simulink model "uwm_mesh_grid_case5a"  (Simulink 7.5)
settings: Solver=ode45  StartTime=0.0  StopTime=3.0  RelTol=1e-4
undefined symbols (not defined in the file or in its folder): D1, Delta, dfilt, DiscIntNeverNeededParam, Discrete, no, powergui, steady, ZData
libraries: powerlib x259, powerlib_extras x68, dsparch4 x11
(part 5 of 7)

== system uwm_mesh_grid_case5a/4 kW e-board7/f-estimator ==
  v : Inport
  Constant : Constant  Value=60  OutDataType=fixdt(1, 16)  OutScaling=2^0
  Fcn : Fcn  Expr=sin(2*pi*u[1])
  Filter1 : dsparch4/Biquad Filter  Tag=BlockMethodSubSystem  DialogController=dspdialog.BiquadFilter  DialogControllerArgs=DataTag8  IIRFiltStruct=Direct form II  CoeffSource=Specify via dialog  BiQuadCoeffs=[1 -1.36 1 1 -1.78 0.87;1 1 0 1 -0.85 0]  a0Flag=Warning  IC=0  ICnum=0  ICden=0  denAccumFracLength=30  denProdOutputFracLength=30  secondMemoryFracLength=15  roundingMode=Floor  overflowMode=off  ScaleValues=[0.05;0.23;1]  optimizeScaleValues=on  ScaleValueMode=Specify via input port (g)  scaleValueFracLength=14  FilterSource=Specify via dialog  dfiltObjectName=dfilt.df2tsos([1 0.3 0.4],[1 0.1 0.2])
  Gain : Gain  Gain=1/150  ParameterDataType=fixdt(1, 16)  ParameterScaling=2^0  OutDataType=fixdt(1, 16)  OutScaling=2^0  SampleTime=dt
  Product : Product  OutDataType=fixdt(1, 16)  OutScaling=2^0
  Scope : Scope
  Sum : Sum  Inputs=|++  OutDataType=fixdt(1, 16)  OutScaling=2^0
  modulo discrete integrator : Subsystem  mask{dt=dt}
      mask prompts: dt "sample time"
  w : Outport  OutDataType=fixdt(1, 16)  OutScaling=2^0
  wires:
  Gain/1 -> Product/1
  v/1 -> Gain/1
  Filter1/1 -> Sum/1, Scope/1
  Product/1 -> Filter1/1
  Sum/1 -> w/1, modulo discrete integrator/1(In1)
  modulo discrete integrator/1(Out1) -> Fcn/1
  Constant/1 -> Sum/2
  Fcn/1 -> Product/2

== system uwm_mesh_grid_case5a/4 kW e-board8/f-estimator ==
  v : Inport
  Constant : Constant  Value=60  OutDataType=fixdt(1, 16)  OutScaling=2^0
  Fcn : Fcn  Expr=sin(2*pi*u[1])
  Filter1 : dsparch4/Biquad Filter  Tag=BlockMethodSubSystem  DialogController=dspdialog.BiquadFilter  DialogControllerArgs=DataTag9  IIRFiltStruct=Direct form II  CoeffSource=Specify via dialog  BiQuadCoeffs=[1 -1.36 1 1 -1.78 0.87;1 1 0 1 -0.85 0]  a0Flag=Warning  IC=0  ICnum=0  ICden=0  denAccumFracLength=30  denProdOutputFracLength=30  secondMemoryFracLength=15  roundingMode=Floor  overflowMode=off  ScaleValues=[0.05;0.23;1]  optimizeScaleValues=on  ScaleValueMode=Specify via input port (g)  scaleValueFracLength=14  FilterSource=Specify via dialog  dfiltObjectName=dfilt.df2tsos([1 0.3 0.4],[1 0.1 0.2])
  Gain : Gain  Gain=1/150  ParameterDataType=fixdt(1, 16)  ParameterScaling=2^0  OutDataType=fixdt(1, 16)  OutScaling=2^0  SampleTime=dt
  Product : Product  OutDataType=fixdt(1, 16)  OutScaling=2^0
  Scope : Scope
  Sum : Sum  Inputs=|++  OutDataType=fixdt(1, 16)  OutScaling=2^0
  modulo discrete integrator : Subsystem  mask{dt=dt}
      mask prompts: dt "sample time"
  w : Outport  OutDataType=fixdt(1, 16)  OutScaling=2^0
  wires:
  Gain/1 -> Product/1
  v/1 -> Gain/1
  Filter1/1 -> Sum/1, Scope/1
  Product/1 -> Filter1/1
  Sum/1 -> w/1, modulo discrete integrator/1(In1)
  modulo discrete integrator/1(Out1) -> Fcn/1
  Constant/1 -> Sum/2
  Fcn/1 -> Product/2

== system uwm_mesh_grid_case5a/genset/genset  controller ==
  wr : Inport
  Vabc : Inport  Port=2
  Iabc : Inport  Port=3
  Preq : Inport  Port=4
  Ereq1 : Inport  Port=5
  Gain : Gain  ParameterDataType=fixdt(1, 16)  ParameterScaling=2^0  OutDataType=fixdt(1, 16)  OutScaling=2^0
  P-w droop : Subsystem
  PVQ computation : Subsystem
  Q-E droop : Subsystem
  exciter : Subsystem
  ic_engine gpvernor : Subsystem
  Pmech : Outport
  Vf : Outport  Port=2
  w : Outport  Port=3
  Pmm : Outport  Port=4
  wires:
  P-w droop/1(w) -> w/1, ic_engine gpvernor/3(w)
  PVQ computation/1(P_pu) -> P-w droop/2(P), ic_engine gpvernor/2(Pmeas)
  PVQ computation/3(Q_pu) -> Q-E droop/2(Q)
  Q-E droop/1(Vpk) -> exciter/2(Ef_mcd_wr)
  ic_engine gpvernor/1(Pmech) -> Pmech/1
  Vabc/1 -> PVQ computation/1(Vabc)
  Iabc/1 -> PVQ computation/2(Iabc)
  exciter/1(Ef) -> Vf/1
  Preq/1 -> P-w droop/1(P_req)
  Ereq1/1 -> Q-E droop/3(E_req)
  PVQ computation/2(Vt) -> Q-E droop/1(v_meas)
  Gain/1 -> ic_engine gpvernor/1(wr), exciter/1(wr)
  wr/1 -> Gain/1
  P-w droop/2(Pmm) -> Pmm/1

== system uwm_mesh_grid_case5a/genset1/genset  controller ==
  wr : Inport
  Vabc : Inport  Port=2
  Iabc : Inport  Port=3
  Preq : Inport  Port=4
  Ereq1 : Inport  Port=5
  Gain : Gain  ParameterDataType=fixdt(1, 16)  ParameterScaling=2^0  OutDataType=fixdt(1, 16)  OutScaling=2^0
  P-w droop : Subsystem
  PVQ computation : Subsystem
  Q-E droop : Subsystem
  exciter : Subsystem
  ic_engine gpvernor : Subsystem
  Pmech : Outport
  Vf : Outport  Port=2
  w : Outport  Port=3
  Pmm : Outport  Port=4
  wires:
  P-w droop/1(w) -> w/1, ic_engine gpvernor/3(w)
  PVQ computation/1(P_pu) -> P-w droop/2(P), ic_engine gpvernor/2(Pmeas)
  PVQ computation/3(Q_pu) -> Q-E droop/2(Q)
  Q-E droop/1(Vpk) -> exciter/2(Ef_mcd_wr)
  ic_engine gpvernor/1(Pmech) -> Pmech/1
  Vabc/1 -> PVQ computation/1(Vabc)
  Iabc/1 -> PVQ computation/2(Iabc)
  exciter/1(Ef) -> Vf/1
  Preq/1 -> P-w droop/1(P_req)
  Ereq1/1 -> Q-E droop/3(E_req)
  PVQ computation/2(Vt) -> Q-E droop/1(v_meas)
  Gain/1 -> ic_engine gpvernor/1(wr), exciter/1(wr)
  wr/1 -> Gain/1
  P-w droop/2(Pmm) -> Pmm/1

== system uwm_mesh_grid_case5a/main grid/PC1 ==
  Three-Phase Series RLC Branch3 : powerlib/Elements/Three-Phase Series RLC Branch  DialogController=POWERSYS.PowerSysDialog  PhysicalDomain=powersysdomain  SubClassName=unknown  LeftPortType=p1  RightPortType=p1  LConnTagsString=A|B|C  RConnTagsString=A|B|C  BranchType=RL  Resistance=R  Inductance=L  Capacitance=1/(336*2*pi*60)  Measurements=None
  A* : PMIOPort  Tag=PMCPort  Port=1  Side=Right
  B* : PMIOPort  Tag=PMCPort  Port=2  Side=Right
  C* : PMIOPort  Tag=PMCPort  Port=3  Side=Right
  A : PMIOPort  Tag=PMCPort  Port=4  Side=Left
  B : PMIOPort  Tag=PMCPort  Port=5  Side=Left
  C : PMIOPort  Tag=PMCPort  Port=6  Side=Left
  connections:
  A*/RConn1 -- Three-Phase Series RLC Branch3/LConn1
  B*/RConn1 -- Three-Phase Series RLC Branch3/LConn2
  C*/RConn1 -- Three-Phase Series RLC Branch3/LConn3
  Three-Phase Series RLC Branch3/RConn1 -- A/RConn1
  Three-Phase Series RLC Branch3/RConn2 -- B/RConn1
  Three-Phase Series RLC Branch3/RConn3 -- C/RConn1

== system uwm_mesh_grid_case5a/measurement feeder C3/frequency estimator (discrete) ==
  v : Inport
  Constant : Constant  Value=60  OutDataType=fixdt(1, 16)  OutScaling=2^0
  Fcn : Fcn  Expr=sin(2*pi*u[1])
  Filter1 : dsparch4/Biquad Filter  Tag=BlockMethodSubSystem  DialogController=dspdialog.BiquadFilter  DialogControllerArgs=DataTag10  IIRFiltStruct=Direct form II  CoeffSource=Specify via dialog  BiQuadCoeffs=[1 -1.36 1 1 -1.78 0.87;1 1 0 1 -0.85 0]  a0Flag=Warning  IC=0  ICnum=0  ICden=0  denAccumFracLength=30  denProdOutputFracLength=30  secondMemoryFracLength=15  roundingMode=Floor  overflowMode=off  ScaleValues=[0.05;0.23;1]  optimizeScaleValues=on  ScaleValueMode=Specify via input port (g)  scaleValueFracLength=14  FilterSource=Specify via dialog  dfiltObjectName=dfilt.df2tsos([1 0.3 0.4],[1 0.1 0.2])
  Gain : Gain  Gain=1/150  ParameterDataType=fixdt(1, 16)  ParameterScaling=2^0  OutDataType=fixdt(1, 16)  OutScaling=2^0  SampleTime=dt
  Product : Product  OutDataType=fixdt(1, 16)  OutScaling=2^0
  Scope : Scope
  Sum : Sum  Inputs=|++  OutDataType=fixdt(1, 16)  OutScaling=2^0
  modulo discrete integrator : Subsystem  mask{dt=dt}
      mask prompts: dt "sample time"
  w : Outport  OutDataType=fixdt(1, 16)  OutScaling=2^0
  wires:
  Fcn/1 -> Product/2
  Constant/1 -> Sum/2
  modulo discrete integrator/1(Out1) -> Fcn/1
  Sum/1 -> modulo discrete integrator/1(In1), w/1
  Product/1 -> Filter1/1
  Filter1/1 -> Scope/1, Sum/1
  v/1 -> Gain/1
  Gain/1 -> Product/1

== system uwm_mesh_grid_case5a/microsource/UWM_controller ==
  note: P
  note: Q
  v_meas : Inport
  i_meas : Inport  Port=2
  E_req : Inport  Port=3
  P_req : Inport  Port=4
  " pu convert P" : Gain  Gain=1/Sbase  ParameterDataType=sfix(16)  ParameterScaling=2^0  OutDataType=sfix(16)  OutScaling=2^0
  " pu convert S" : Gain  Gain=1/Sbase  ParameterDataType=sfix(16)  ParameterScaling=2^0  OutDataType=sfix(16)  OutScaling=2^0
  " pu convert V" : Gain  Gain=1/(Vbase/sqrt(3))  ParameterDataType=sfix(16)  ParameterScaling=2^0  OutDataType=sfix(16)  OutScaling=2^0
  3-phase  Instantaneous  Active & Reactive Power : powerlib_extras/Measurements/3-phase  Instantaneous  Active & Reactive Power  DialogController=POWERSYS.PowerSysDialog  SystemSampleTime=-1
  Demux : Demux  Outputs=2
  PI-Control : Subsystem
  RMS : Fcn  Expr=sqrt(u(1)*u(1)+u(2)*u(2)+u(3)*u(3))/sqrt(3)
  Sum : Sum  Inputs=|-+  OutDataType=sfix(16)  OutScaling=2^0
  Sum1 : Sum  Inputs=|+-  OutDataType=sfix(16)  OutScaling=2^0
  Sum2 : Sum  Inputs=+-|  OutDataType=sfix(16)  OutScaling=2^0
  Sum3 : Sum  Inputs=+++  OutDataType=sfix(16)  OutScaling=2^0
  Transfer Fcn : TransferFcn  Denominator=[.01 1]
  Transfer Fcn1 : TransferFcn  Denominator=[.01 1]
  Transfer Fcn2 : TransferFcn  Denominator=[.01 1]
  k : Gain  Gain=1/pi  ParameterDataType=sfix(16)  ParameterScaling=2^0  OutDataType=sfix(16)  OutScaling=2^0
  limiter : Subsystem
  mP droop : Gain  Gain=pi  ParameterDataType=sfix(16)  ParameterScaling=2^0  OutDataType=sfix(16)  OutScaling=2^0
  "mQ droop " : Gain  Gain=0.05  ParameterDataType=sfix(16)  ParameterScaling=2^0  OutDataType=sfix(16)  OutScaling=2^0
  w0 : Constant  Value=60*2*pi  OutDataType=fixdt(1, 16)  OutScaling=2^0
  Vpk : Outport
  w : Outport  Port=2
  Pmm : Outport  Port=3
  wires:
  Transfer Fcn2/1 -> " pu convert V"/1
  Transfer Fcn/1 -> " pu convert P"/1
  " pu convert P"/1 -> "mQ droop "/1
  Transfer Fcn1/1 -> " pu convert S"/1
  " pu convert S"/1 -> limiter/1(In1), Sum2/2
  i_meas/1 -> 3-phase  Instantaneous  Active & Reactive Power/2
  P_req/1 -> Sum2/1
  mP droop/1 -> Sum3/2
  limiter/1(Out1) -> Sum3/1, k/1
  w0/1 -> Sum3/3
  Sum2/1 -> mP droop/1
  Sum1/1 -> PI-Control/1(In1)
  Sum/1 -> Sum1/1
  "mQ droop "/1 -> Sum/1
  RMS/1 -> Transfer Fcn2/1
  Demux/2 -> Transfer Fcn/1
  Demux/1 -> Transfer Fcn1/1
  3-phase  Instantaneous  Active & Reactive Power/1 -> Demux/1
  v_meas/1 -> RMS/1, 3-phase  Instantaneous  Active & Reactive Power/1
  PI-Control/1(Out1) -> Vpk/1
  Sum3/1 -> w/1
  E_req/1 -> Sum/2
  " pu convert V"/1 -> Sum1/2
  k/1 -> Pmm/1

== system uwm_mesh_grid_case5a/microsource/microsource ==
  Vpk : Inport  OutDataType=fixdt(1, 16)  OutScaling=2^0
  w : Inport  Port=2  OutDataType=fixdt(1, 16)  OutScaling=2^0
  Demux : Demux  Outputs=3
  Ground2 : powerlib/Elements/Ground  DialogController=POWERSYS.PowerSysDialog  PhysicalDomain=powersysdomain  SubClassName=unknown  LeftPortType=p1  RightPortType=p1  LConnTagsString=a
  Integrator : Integrator
  Mux : Mux  Inputs=3
  Product : Product  OutDataType=sfix(16)  OutScaling=2^0
  Series RLC Branch : powerlib/Elements/Series RLC Branch  DialogController=POWERSYS.PowerSysDialog  PhysicalDomain=powersysdomain  SubClassName=unknown  LeftPortType=p1  RightPortType=p1  LConnTagsString=__new0  RConnTagsString=__new0  BranchType=C  Resistance=1  Inductance=1e-3  SetiL0=off  InitialCurrent=0  Capacitance=1e-8  Setx0=off  InitialVoltage=0  Measurements=None
  phaseA : powerlib/Electrical Sources/Controlled Voltage Source  DialogController=POWERSYS.PowerSysDialog  SystemSampleTime=-1  Initialize=on  Source_Type=AC  Amplitude=0  Phase=0  Frequency=0  Measurements=None
  phaseB : powerlib/Electrical Sources/Controlled Voltage Source  DialogController=POWERSYS.PowerSysDialog  SystemSampleTime=-1  Initialize=on  Source_Type=AC  Amplitude=0  Phase=0  Frequency=0  Measurements=None
  phaseC : powerlib/Electrical Sources/Controlled Voltage Source  DialogController=POWERSYS.PowerSysDialog  SystemSampleTime=-1  Initialize=on  Source_Type=AC  Amplitude=0  Phase=0  Frequency=0  Measurements=None
  v_A : Fcn  Expr=cos(u)
  v_B : Fcn  Expr=cos(u-2*pi/3)
  v_C : Fcn  Expr=cos(u+2*pi/3)
  Va : PMIOPort  Tag=PMCPort  Port=1  Side=Right
  Vb : PMIOPort  Tag=PMCPort  Port=2  Side=Right
  Vc : PMIOPort  Tag=PMCPort  Port=3  Side=Right
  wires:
  Product/1 -> Demux/1
  Vpk/1 -> Product/1
  Mux/1 -> Product/2
  w/1 -> Integrator/1
  Integrator/1 -> v_A/1, v_B/1, v_C/1
  v_A/1 -> Mux/1
  v_B/1 -> Mux/2
  v_C/1 -> Mux/3
  Demux/1 -> phaseA/1
  Demux/2 -> phaseB/1
  Demux/3 -> phaseC/1
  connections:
  Vb/RConn1 -- phaseB/RConn1 -- phaseA/LConn1
  Va/RConn1 -- phaseC/LConn1 -- phaseA/RConn1
  Vc/RConn1 -- phaseC/RConn1
  Series RLC Branch/RConn1 -- Ground2/LConn1
  Series RLC Branch/LConn1 -- phaseB/LConn1

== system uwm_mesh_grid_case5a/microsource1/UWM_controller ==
  note: P
  note: Q
  v_meas : Inport
  i_meas : Inport  Port=2
  E_req : Inport  Port=3
  P_req : Inport  Port=4
  " pu convert P" : Gain  Gain=1/Sbase  ParameterDataType=sfix(16)  ParameterScaling=2^0  OutDataType=sfix(16)  OutScaling=2^0
  " pu convert S" : Gain  Gain=1/Sbase  ParameterDataType=sfix(16)  ParameterScaling=2^0  OutDataType=sfix(16)  OutScaling=2^0
  " pu convert V" : Gain  Gain=1/(Vbase/sqrt(3))  ParameterDataType=sfix(16)  ParameterScaling=2^0  OutDataType=sfix(16)  OutScaling=2^0
  3-phase  Instantaneous  Active & Reactive Power : powerlib_extras/Measurements/3-phase  Instantaneous  Active & Reactive Power  DialogController=POWERSYS.PowerSysDialog  SystemSampleTime=-1
  Demux : Demux  Outputs=2
  PI-Control : Subsystem
  RMS : Fcn  Expr=sqrt(u(1)*u(1)+u(2)*u(2)+u(3)*u(3))/sqrt(3)
  Sum : Sum  Inputs=|-+  OutDataType=sfix(16)  OutScaling=2^0
  Sum1 : Sum  Inputs=|+-  OutDataType=sfix(16)  OutScaling=2^0
  Sum2 : Sum  Inputs=+-|  OutDataType=sfix(16)  OutScaling=2^0
  Sum3 : Sum  Inputs=+++  OutDataType=sfix(16)  OutScaling=2^0
  Transfer Fcn : TransferFcn  Denominator=[.01 1]
  Transfer Fcn1 : TransferFcn  Denominator=[.01 1]
  Transfer Fcn2 : TransferFcn  Denominator=[.01 1]
  k : Gain  Gain=1/pi  ParameterDataType=sfix(16)  ParameterScaling=2^0  OutDataType=sfix(16)  OutScaling=2^0
  limiter : Subsystem
  mP droop : Gain  Gain=pi  ParameterDataType=sfix(16)  ParameterScaling=2^0  OutDataType=sfix(16)  OutScaling=2^0
  "mQ droop " : Gain  Gain=0.05  ParameterDataType=sfix(16)  ParameterScaling=2^0  OutDataType=sfix(16)  OutScaling=2^0
  w0 : Constant  Value=60*2*pi  OutDataType=fixdt(1, 16)  OutScaling=2^0
  Vpk : Outport
  w : Outport  Port=2
  Pmm : Outport  Port=3
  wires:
  Transfer Fcn2/1 -> " pu convert V"/1
  Transfer Fcn/1 -> " pu convert P"/1
  " pu convert P"/1 -> "mQ droop "/1
  Transfer Fcn1/1 -> " pu convert S"/1
  " pu convert S"/1 -> limiter/1(In1), Sum2/2
  i_meas/1 -> 3-phase  Instantaneous  Active & Reactive Power/2
  P_req/1 -> Sum2/1
  mP droop/1 -> Sum3/2
  limiter/1(Out1) -> Sum3/1, k/1
  w0/1 -> Sum3/3
  Sum2/1 -> mP droop/1
  Sum1/1 -> PI-Control/1(In1)
  Sum/1 -> Sum1/1
  "mQ droop "/1 -> Sum/1
  RMS/1 -> Transfer Fcn2/1
  Demux/2 -> Transfer Fcn/1
  Demux/1 -> Transfer Fcn1/1
  3-phase  Instantaneous  Active & Reactive Power/1 -> Demux/1
  v_meas/1 -> RMS/1, 3-phase  Instantaneous  Active & Reactive Power/1
  PI-Control/1(Out1) -> Vpk/1
  Sum3/1 -> w/1
  E_req/1 -> Sum/2
  " pu convert V"/1 -> Sum1/2
  k/1 -> Pmm/1

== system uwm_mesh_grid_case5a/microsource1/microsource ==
  Vpk : Inport  OutDataType=fixdt(1, 16)  OutScaling=2^0
  w : Inport  Port=2  OutDataType=fixdt(1, 16)  OutScaling=2^0
  Demux : Demux  Outputs=3
  Ground2 : powerlib/Elements/Ground  DialogController=POWERSYS.PowerSysDialog  PhysicalDomain=powersysdomain  SubClassName=unknown  LeftPortType=p1  RightPortType=p1  LConnTagsString=a
  Integrator : Integrator
  Mux : Mux  Inputs=3
  Product : Product  OutDataType=sfix(16)  OutScaling=2^0
  Series RLC Branch : powerlib/Elements/Series RLC Branch  DialogController=POWERSYS.PowerSysDialog  PhysicalDomain=powersysdomain  SubClassName=unknown  LeftPortType=p1  RightPortType=p1  LConnTagsString=__new0  RConnTagsString=__new0  BranchType=C  Resistance=1  Inductance=1e-3  SetiL0=off  InitialCurrent=0  Capacitance=1e-8  Setx0=off  InitialVoltage=0  Measurements=None
  phaseA : powerlib/Electrical Sources/Controlled Voltage Source  DialogController=POWERSYS.PowerSysDialog  SystemSampleTime=-1  Initialize=on  Source_Type=AC  Amplitude=0  Phase=0  Frequency=0  Measurements=None
  phaseB : powerlib/Electrical Sources/Controlled Voltage Source  DialogController=POWERSYS.PowerSysDialog  SystemSampleTime=-1  Initialize=on  Source_Type=AC  Amplitude=0  Phase=0  Frequency=0  Measurements=None
  phaseC : powerlib/Electrical Sources/Controlled Voltage Source  DialogController=POWERSYS.PowerSysDialog  SystemSampleTime=-1  Initialize=on  Source_Type=AC  Amplitude=0  Phase=0  Frequency=0  Measurements=None
  v_A : Fcn  Expr=cos(u)
  v_B : Fcn  Expr=cos(u-2*pi/3)
  v_C : Fcn  Expr=cos(u+2*pi/3)
  Va : PMIOPort  Tag=PMCPort  Port=1  Side=Right
  Vb : PMIOPort  Tag=PMCPort  Port=2  Side=Right
  Vc : PMIOPort  Tag=PMCPort  Port=3  Side=Right
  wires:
  Product/1 -> Demux/1
  Vpk/1 -> Product/1
  Mux/1 -> Product/2
  w/1 -> Integrator/1
  Integrator/1 -> v_A/1, v_B/1, v_C/1
  v_A/1 -> Mux/1
  v_B/1 -> Mux/2
  v_C/1 -> Mux/3
  Demux/1 -> phaseA/1
  Demux/2 -> phaseB/1
  Demux/3 -> phaseC/1
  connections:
  Vb/RConn1 -- phaseB/RConn1 -- phaseA/LConn1
  Va/RConn1 -- phaseC/LConn1 -- phaseA/RConn1
  Vc/RConn1 -- phaseC/RConn1
  Series RLC Branch/RConn1 -- Ground2/LConn1
  Series RLC Branch/LConn1 -- phaseB/LConn1

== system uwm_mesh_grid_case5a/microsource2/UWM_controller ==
  note: P
  note: Q
  v_meas : Inport
  i_meas : Inport  Port=2
  E_req : Inport  Port=3
  P_req : Inport  Port=4
  " pu convert P" : Gain  Gain=1/Sbase  ParameterDataType=sfix(16)  ParameterScaling=2^0  OutDataType=sfix(16)  OutScaling=2^0
  " pu convert S" : Gain  Gain=1/Sbase  ParameterDataType=sfix(16)  ParameterScaling=2^0  OutDataType=sfix(16)  OutScaling=2^0
  " pu convert V" : Gain  Gain=1/(Vbase/sqrt(3))  ParameterDataType=sfix(16)  ParameterScaling=2^0  OutDataType=sfix(16)  OutScaling=2^0
  3-phase  Instantaneous  Active & Reactive Power : powerlib_extras/Measurements/3-phase  Instantaneous  Active & Reactive Power  DialogController=POWERSYS.PowerSysDialog  SystemSampleTime=-1
  Demux : Demux  Outputs=2
  PI-Control : Subsystem
  RMS : Fcn  Expr=sqrt(u(1)*u(1)+u(2)*u(2)+u(3)*u(3))/sqrt(3)
  Sum : Sum  Inputs=|-+  OutDataType=sfix(16)  OutScaling=2^0
  Sum1 : Sum  Inputs=|+-  OutDataType=sfix(16)  OutScaling=2^0
  Sum2 : Sum  Inputs=+-|  OutDataType=sfix(16)  OutScaling=2^0
  Sum3 : Sum  Inputs=+++  OutDataType=sfix(16)  OutScaling=2^0
  Transfer Fcn : TransferFcn  Denominator=[.01 1]
  Transfer Fcn1 : TransferFcn  Denominator=[.01 1]
  Transfer Fcn2 : TransferFcn  Denominator=[.01 1]
  k : Gain  Gain=1/pi  ParameterDataType=sfix(16)  ParameterScaling=2^0  OutDataType=sfix(16)  OutScaling=2^0
  limiter : Subsystem
  mP droop : Gain  Gain=pi  ParameterDataType=sfix(16)  ParameterScaling=2^0  OutDataType=sfix(16)  OutScaling=2^0
  "mQ droop " : Gain  Gain=0.05  ParameterDataType=sfix(16)  ParameterScaling=2^0  OutDataType=sfix(16)  OutScaling=2^0
  w0 : Constant  Value=60*2*pi  OutDataType=fixdt(1, 16)  OutScaling=2^0
  Vpk : Outport
  w : Outport  Port=2
  Pmm : Outport  Port=3
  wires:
  Transfer Fcn2/1 -> " pu convert V"/1
  Transfer Fcn/1 -> " pu convert P"/1
  " pu convert P"/1 -> "mQ droop "/1
  Transfer Fcn1/1 -> " pu convert S"/1
  " pu convert S"/1 -> limiter/1(In1), Sum2/2
  i_meas/1 -> 3-phase  Instantaneous  Active & Reactive Power/2
  P_req/1 -> Sum2/1
  mP droop/1 -> Sum3/2
  limiter/1(Out1) -> Sum3/1, k/1
  w0/1 -> Sum3/3
  Sum2/1 -> mP droop/1
  Sum1/1 -> PI-Control/1(In1)
  Sum/1 -> Sum1/1
  "mQ droop "/1 -> Sum/1
  RMS/1 -> Transfer Fcn2/1
  Demux/2 -> Transfer Fcn/1
  Demux/1 -> Transfer Fcn1/1
  3-phase  Instantaneous  Active & Reactive Power/1 -> Demux/1
  v_meas/1 -> RMS/1, 3-phase  Instantaneous  Active & Reactive Power/1
  PI-Control/1(Out1) -> Vpk/1
  Sum3/1 -> w/1
  E_req/1 -> Sum/2
  " pu convert V"/1 -> Sum1/2
  k/1 -> Pmm/1

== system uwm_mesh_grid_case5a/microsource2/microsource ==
  Vpk : Inport  OutDataType=fixdt(1, 16)  OutScaling=2^0
  w : Inport  Port=2  OutDataType=fixdt(1, 16)  OutScaling=2^0
  Demux : Demux  Outputs=3
  Ground2 : powerlib/Elements/Ground  DialogController=POWERSYS.PowerSysDialog  PhysicalDomain=powersysdomain  SubClassName=unknown  LeftPortType=p1  RightPortType=p1  LConnTagsString=a
  Integrator : Integrator
  Mux : Mux  Inputs=3
  Product : Product  OutDataType=sfix(16)  OutScaling=2^0
  Series RLC Branch : powerlib/Elements/Series RLC Branch  DialogController=POWERSYS.PowerSysDialog  PhysicalDomain=powersysdomain  SubClassName=unknown  LeftPortType=p1  RightPortType=p1  LConnTagsString=__new0  RConnTagsString=__new0  BranchType=C  Resistance=1  Inductance=1e-3  SetiL0=off  InitialCurrent=0  Capacitance=1e-8  Setx0=off  InitialVoltage=0  Measurements=None
  phaseA : powerlib/Electrical Sources/Controlled Voltage Source  DialogController=POWERSYS.PowerSysDialog  SystemSampleTime=-1  Initialize=on  Source_Type=AC  Amplitude=0  Phase=0  Frequency=0  Measurements=None
  phaseB : powerlib/Electrical Sources/Controlled Voltage Source  DialogController=POWERSYS.PowerSysDialog  SystemSampleTime=-1  Initialize=on  Source_Type=AC  Amplitude=0  Phase=0  Frequency=0  Measurements=None
  phaseC : powerlib/Electrical Sources/Controlled Voltage Source  DialogController=POWERSYS.PowerSysDialog  SystemSampleTime=-1  Initialize=on  Source_Type=AC  Amplitude=0  Phase=0  Frequency=0  Measurements=None
  v_A : Fcn  Expr=cos(u)
  v_B : Fcn  Expr=cos(u-2*pi/3)
  v_C : Fcn  Expr=cos(u+2*pi/3)
  Va : PMIOPort  Tag=PMCPort  Port=1  Side=Right
  Vb : PMIOPort  Tag=PMCPort  Port=2  Side=Right
  Vc : PMIOPort  Tag=PMCPort  Port=3  Side=Right
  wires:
  Product/1 -> Demux/1
  Vpk/1 -> Product/1
  Mux/1 -> Product/2
  w/1 -> Integrator/1
  Integrator/1 -> v_A/1, v_B/1, v_C/1
  v_A/1 -> Mux/1
  v_B/1 -> Mux/2
  v_C/1 -> Mux/3
  Demux/1 -> phaseA/1
  Demux/2 -> phaseB/1
  Demux/3 -> phaseC/1
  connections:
  Vb/RConn1 -- phaseB/RConn1 -- phaseA/LConn1
  Va/RConn1 -- phaseC/LConn1 -- phaseA/RConn1
  Vc/RConn1 -- phaseC/RConn1
  Series RLC Branch/RConn1 -- Ground2/LConn1
  Series RLC Branch/LConn1 -- phaseB/LConn1

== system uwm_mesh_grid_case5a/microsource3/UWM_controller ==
  note: P
  note: Q
  v_meas : Inport
  i_meas : Inport  Port=2
  E_req : Inport  Port=3
  P_req : Inport  Port=4
  " pu convert P" : Gain  Gain=1/Sbase  ParameterDataType=sfix(16)  ParameterScaling=2^0  OutDataType=sfix(16)  OutScaling=2^0
  " pu convert S" : Gain  Gain=1/Sbase  ParameterDataType=sfix(16)  ParameterScaling=2^0  OutDataType=sfix(16)  OutScaling=2^0
  " pu convert V" : Gain  Gain=1/(Vbase/sqrt(3))  ParameterDataType=sfix(16)  ParameterScaling=2^0  OutDataType=sfix(16)  OutScaling=2^0
  3-phase  Instantaneous  Active & Reactive Power : powerlib_extras/Measurements/3-phase  Instantaneous  Active & Reactive Power  DialogController=POWERSYS.PowerSysDialog  SystemSampleTime=-1
  Demux : Demux  Outputs=2
  PI-Control : Subsystem
  RMS : Fcn  Expr=sqrt(u(1)*u(1)+u(2)*u(2)+u(3)*u(3))/sqrt(3)
  Sum : Sum  Inputs=|-+  OutDataType=sfix(16)  OutScaling=2^0
  Sum1 : Sum  Inputs=|+-  OutDataType=sfix(16)  OutScaling=2^0
  Sum2 : Sum  Inputs=+-|  OutDataType=sfix(16)  OutScaling=2^0
  Sum3 : Sum  Inputs=+++  OutDataType=sfix(16)  OutScaling=2^0
  Transfer Fcn : TransferFcn  Denominator=[.01 1]
  Transfer Fcn1 : TransferFcn  Denominator=[.01 1]
  Transfer Fcn2 : TransferFcn  Denominator=[.01 1]
  k : Gain  Gain=1/pi  ParameterDataType=sfix(16)  ParameterScaling=2^0  OutDataType=sfix(16)  OutScaling=2^0
  limiter : Subsystem
  mP droop : Gain  Gain=pi  ParameterDataType=sfix(16)  ParameterScaling=2^0  OutDataType=sfix(16)  OutScaling=2^0
  "mQ droop " : Gain  Gain=0.05  ParameterDataType=sfix(16)  ParameterScaling=2^0  OutDataType=sfix(16)  OutScaling=2^0
  w0 : Constant  Value=60*2*pi  OutDataType=fixdt(1, 16)  OutScaling=2^0
  Vpk : Outport
  w : Outport  Port=2
  Pmm : Outport  Port=3
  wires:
  Transfer Fcn2/1 -> " pu convert V"/1
  Transfer Fcn/1 -> " pu convert P"/1
  " pu convert P"/1 -> "mQ droop "/1
  Transfer Fcn1/1 -> " pu convert S"/1
  " pu convert S"/1 -> limiter/1(In1), Sum2/2
  i_meas/1 -> 3-phase  Instantaneous  Active & Reactive Power/2
  P_req/1 -> Sum2/1
  mP droop/1 -> Sum3/2
  limiter/1(Out1) -> Sum3/1, k/1
  w0/1 -> Sum3/3
  Sum2/1 -> mP droop/1
  Sum1/1 -> PI-Control/1(In1)
  Sum/1 -> Sum1/1
  "mQ droop "/1 -> Sum/1
  RMS/1 -> Transfer Fcn2/1
  Demux/2 -> Transfer Fcn/1
  Demux/1 -> Transfer Fcn1/1
  3-phase  Instantaneous  Active & Reactive Power/1 -> Demux/1
  v_meas/1 -> RMS/1, 3-phase  Instantaneous  Active & Reactive Power/1
  PI-Control/1(Out1) -> Vpk/1
  Sum3/1 -> w/1
  E_req/1 -> Sum/2
  " pu convert V"/1 -> Sum1/2
  k/1 -> Pmm/1

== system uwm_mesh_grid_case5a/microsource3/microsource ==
  Vpk : Inport  OutDataType=fixdt(1, 16)  OutScaling=2^0
  w : Inport  Port=2  OutDataType=fixdt(1, 16)  OutScaling=2^0
  Demux : Demux  Outputs=3
  Ground2 : powerlib/Elements/Ground  DialogController=POWERSYS.PowerSysDialog  PhysicalDomain=powersysdomain  SubClassName=unknown  LeftPortType=p1  RightPortType=p1  LConnTagsString=a
  Integrator : Integrator
  Mux : Mux  Inputs=3
  Product : Product  OutDataType=sfix(16)  OutScaling=2^0
  Series RLC Branch : powerlib/Elements/Series RLC Branch  DialogController=POWERSYS.PowerSysDialog  PhysicalDomain=powersysdomain  SubClassName=unknown  LeftPortType=p1  RightPortType=p1  LConnTagsString=__new0  RConnTagsString=__new0  BranchType=C  Resistance=1  Inductance=1e-3  SetiL0=off  InitialCurrent=0  Capacitance=1e-8  Setx0=off  InitialVoltage=0  Measurements=None
  phaseA : powerlib/Electrical Sources/Controlled Voltage Source  DialogController=POWERSYS.PowerSysDialog  SystemSampleTime=-1  Initialize=on  Source_Type=AC  Amplitude=0  Phase=0  Frequency=0  Measurements=None
  phaseB : powerlib/Electrical Sources/Controlled Voltage Source  DialogController=POWERSYS.PowerSysDialog  SystemSampleTime=-1  Initialize=on  Source_Type=AC  Amplitude=0  Phase=0  Frequency=0  Measurements=None
  phaseC : powerlib/Electrical Sources/Controlled Voltage Source  DialogController=POWERSYS.PowerSysDialog  SystemSampleTime=-1  Initialize=on  Source_Type=AC  Amplitude=0  Phase=0  Frequency=0  Measurements=None
  v_A : Fcn  Expr=cos(u)
  v_B : Fcn  Expr=cos(u-2*pi/3)
  v_C : Fcn  Expr=cos(u+2*pi/3)
  Va : PMIOPort  Tag=PMCPort  Port=1  Side=Right
  Vb : PMIOPort  Tag=PMCPort  Port=2  Side=Right
  Vc : PMIOPort  Tag=PMCPort  Port=3  Side=Right
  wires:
  Product/1 -> Demux/1
  Vpk/1 -> Product/1
  Mux/1 -> Product/2
  w/1 -> Integrator/1
  Integrator/1 -> v_A/1, v_B/1, v_C/1
  v_A/1 -> Mux/1
  v_B/1 -> Mux/2
  v_C/1 -> Mux/3
  Demux/1 -> phaseA/1
  Demux/2 -> phaseB/1
  Demux/3 -> phaseC/1
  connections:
  Vb/RConn1 -- phaseB/RConn1 -- phaseA/LConn1
  Va/RConn1 -- phaseC/LConn1 -- phaseA/RConn1
  Vc/RConn1 -- phaseC/RConn1
  Series RLC Branch/RConn1 -- Ground2/LConn1
  Series RLC Branch/LConn1 -- phaseB/LConn1

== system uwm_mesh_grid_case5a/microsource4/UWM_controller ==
  note: P
  note: Q
  v_meas : Inport
  i_meas : Inport  Port=2
  E_req : Inport  Port=3
  P_req : Inport  Port=4
  " pu convert P" : Gain  Gain=1/Sbase  ParameterDataType=sfix(16)  ParameterScaling=2^0  OutDataType=sfix(16)  OutScaling=2^0
  " pu convert S" : Gain  Gain=1/Sbase  ParameterDataType=sfix(16)  ParameterScaling=2^0  OutDataType=sfix(16)  OutScaling=2^0
  " pu convert V" : Gain  Gain=1/(Vbase/sqrt(3))  ParameterDataType=sfix(16)  ParameterScaling=2^0  OutDataType=sfix(16)  OutScaling=2^0
  3-phase  Instantaneous  Active & Reactive Power : powerlib_extras/Measurements/3-phase  Instantaneous  Active & Reactive Power  DialogController=POWERSYS.PowerSysDialog  SystemSampleTime=-1
  Demux : Demux  Outputs=2
  PI-Control : Subsystem
  RMS : Fcn  Expr=sqrt(u(1)*u(1)+u(2)*u(2)+u(3)*u(3))/sqrt(3)
  Sum : Sum  Inputs=|-+  OutDataType=sfix(16)  OutScaling=2^0
  Sum1 : Sum  Inputs=|+-  OutDataType=sfix(16)  OutScaling=2^0
  Sum2 : Sum  Inputs=+-|  OutDataType=sfix(16)  OutScaling=2^0
  Sum3 : Sum  Inputs=+++  OutDataType=sfix(16)  OutScaling=2^0
  Transfer Fcn : TransferFcn  Denominator=[.01 1]
  Transfer Fcn1 : TransferFcn  Denominator=[.01 1]
  Transfer Fcn2 : TransferFcn  Denominator=[.01 1]
  k : Gain  Gain=1/pi  ParameterDataType=sfix(16)  ParameterScaling=2^0  OutDataType=sfix(16)  OutScaling=2^0
  limiter : Subsystem
  mP droop : Gain  Gain=pi  ParameterDataType=sfix(16)  ParameterScaling=2^0  OutDataType=sfix(16)  OutScaling=2^0
  "mQ droop " : Gain  Gain=0.05  ParameterDataType=sfix(16)  ParameterScaling=2^0  OutDataType=sfix(16)  OutScaling=2^0
  w0 : Constant  Value=60*2*pi  OutDataType=fixdt(1, 16)  OutScaling=2^0
  Vpk : Outport
  w : Outport  Port=2
  Pmm : Outport  Port=3
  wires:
  Transfer Fcn2/1 -> " pu convert V"/1
  Transfer Fcn/1 -> " pu convert P"/1
  " pu convert P"/1 -> "mQ droop "/1
  Transfer Fcn1/1 -> " pu convert S"/1
  " pu convert S"/1 -> limiter/1(In1), Sum2/2
  i_meas/1 -> 3-phase  Instantaneous  Active & Reactive Power/2
  P_req/1 -> Sum2/1
  mP droop/1 -> Sum3/2
  limiter/1(Out1) -> Sum3/1, k/1
  w0/1 -> Sum3/3
  Sum2/1 -> mP droop/1
  Sum1/1 -> PI-Control/1(In1)
  Sum/1 -> Sum1/1
  "mQ droop "/1 -> Sum/1
  RMS/1 -> Transfer Fcn2/1
  Demux/2 -> Transfer Fcn/1
  Demux/1 -> Transfer Fcn1/1
  3-phase  Instantaneous  Active & Reactive Power/1 -> Demux/1
  v_meas/1 -> RMS/1, 3-phase  Instantaneous  Active & Reactive Power/1
  PI-Control/1(Out1) -> Vpk/1
  Sum3/1 -> w/1
  E_req/1 -> Sum/2
  " pu convert V"/1 -> Sum1/2
  k/1 -> Pmm/1

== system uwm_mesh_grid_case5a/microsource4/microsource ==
  Vpk : Inport  OutDataType=fixdt(1, 16)  OutScaling=2^0
  w : Inport  Port=2  OutDataType=fixdt(1, 16)  OutScaling=2^0
  Demux : Demux  Outputs=3
  Ground2 : powerlib/Elements/Ground  DialogController=POWERSYS.PowerSysDialog  PhysicalDomain=powersysdomain  SubClassName=unknown  LeftPortType=p1  RightPortType=p1  LConnTagsString=a
  Integrator : Integrator
  Mux : Mux  Inputs=3
  Product : Product  OutDataType=sfix(16)  OutScaling=2^0
  Series RLC Branch : powerlib/Elements/Series RLC Branch  DialogController=POWERSYS.PowerSysDialog  PhysicalDomain=powersysdomain  SubClassName=unknown  LeftPortType=p1  RightPortType=p1  LConnTagsString=__new0  RConnTagsString=__new0  BranchType=C  Resistance=1  Inductance=1e-3  SetiL0=off  InitialCurrent=0  Capacitance=1e-8  Setx0=off  InitialVoltage=0  Measurements=None
  phaseA : powerlib/Electrical Sources/Controlled Voltage Source  DialogController=POWERSYS.PowerSysDialog  SystemSampleTime=-1  Initialize=on  Source_Type=AC  Amplitude=0  Phase=0  Frequency=0  Measurements=None
  phaseB : powerlib/Electrical Sources/Controlled Voltage Source  DialogController=POWERSYS.PowerSysDialog  SystemSampleTime=-1  Initialize=on  Source_Type=AC  Amplitude=0  Phase=0  Frequency=0  Measurements=None
  phaseC : powerlib/Electrical Sources/Controlled Voltage Source  DialogController=POWERSYS.PowerSysDialog  SystemSampleTime=-1  Initialize=on  Source_Type=AC  Amplitude=0  Phase=0  Frequency=0  Measurements=None
  v_A : Fcn  Expr=cos(u)
  v_B : Fcn  Expr=cos(u-2*pi/3)
  v_C : Fcn  Expr=cos(u+2*pi/3)
  Va : PMIOPort  Tag=PMCPort  Port=1  Side=Right
  Vb : PMIOPort  Tag=PMCPort  Port=2  Side=Right
  Vc : PMIOPort  Tag=PMCPort  Port=3  Side=Right
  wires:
  Product/1 -> Demux/1
  Vpk/1 -> Product/1
  Mux/1 -> Product/2
  w/1 -> Integrator/1
  Integrator/1 -> v_A/1, v_B/1, v_C/1
  v_A/1 -> Mux/1
  v_B/1 -> Mux/2
  v_C/1 -> Mux/3
  Demux/1 -> phaseA/1
  Demux/2 -> phaseB/1
  Demux/3 -> phaseC/1
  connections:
  Vb/RConn1 -- phaseB/RConn1 -- phaseA/LConn1
  Va/RConn1 -- phaseC/LConn1 -- phaseA/RConn1
  Vc/RConn1 -- phaseC/RConn1
  Series RLC Branch/RConn1 -- Ground2/LConn1
  Series RLC Branch/LConn1 -- phaseB/LConn1

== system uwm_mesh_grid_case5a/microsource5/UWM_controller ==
  note: P
  note: Q
  v_meas : Inport
  i_meas : Inport  Port=2
  E_req : Inport  Port=3
  P_req : Inport  Port=4
  " pu convert P" : Gain  Gain=1/Sbase  ParameterDataType=sfix(16)  ParameterScaling=2^0  OutDataType=sfix(16)  OutScaling=2^0
  " pu convert S" : Gain  Gain=1/Sbase  ParameterDataType=sfix(16)  ParameterScaling=2^0  OutDataType=sfix(16)  OutScaling=2^0
  " pu convert V" : Gain  Gain=1/(Vbase/sqrt(3))  ParameterDataType=sfix(16)  ParameterScaling=2^0  OutDataType=sfix(16)  OutScaling=2^0
  3-phase  Instantaneous  Active & Reactive Power : powerlib_extras/Measurements/3-phase  Instantaneous  Active & Reactive Power  DialogController=POWERSYS.PowerSysDialog  SystemSampleTime=-1
  Demux : Demux  Outputs=2
  PI-Control : Subsystem
  RMS : Fcn  Expr=sqrt(u(1)*u(1)+u(2)*u(2)+u(3)*u(3))/sqrt(3)
  Sum : Sum  Inputs=|-+  OutDataType=sfix(16)  OutScaling=2^0
  Sum1 : Sum  Inputs=|+-  OutDataType=sfix(16)  OutScaling=2^0
  Sum2 : Sum  Inputs=+-|  OutDataType=sfix(16)  OutScaling=2^0
  Sum3 : Sum  Inputs=+++  OutDataType=sfix(16)  OutScaling=2^0
  Transfer Fcn : TransferFcn  Denominator=[.01 1]
  Transfer Fcn1 : TransferFcn  Denominator=[.01 1]
  Transfer Fcn2 : TransferFcn  Denominator=[.01 1]
  k : Gain  Gain=1/pi  ParameterDataType=sfix(16)  ParameterScaling=2^0  OutDataType=sfix(16)  OutScaling=2^0
  limiter : Subsystem
  mP droop : Gain  Gain=pi  ParameterDataType=sfix(16)  ParameterScaling=2^0  OutDataType=sfix(16)  OutScaling=2^0
  "mQ droop " : Gain  Gain=0.05  ParameterDataType=sfix(16)  ParameterScaling=2^0  OutDataType=sfix(16)  OutScaling=2^0
  w0 : Constant  Value=60*2*pi  OutDataType=fixdt(1, 16)  OutScaling=2^0
  Vpk : Outport
  w : Outport  Port=2
  Pmm : Outport  Port=3
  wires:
  Transfer Fcn2/1 -> " pu convert V"/1
  Transfer Fcn/1 -> " pu convert P"/1
  " pu convert P"/1 -> "mQ droop "/1
  Transfer Fcn1/1 -> " pu convert S"/1
  " pu convert S"/1 -> limiter/1(In1), Sum2/2
  i_meas/1 -> 3-phase  Instantaneous  Active & Reactive Power/2
  P_req/1 -> Sum2/1
  mP droop/1 -> Sum3/2
  limiter/1(Out1) -> Sum3/1, k/1
  w0/1 -> Sum3/3
  Sum2/1 -> mP droop/1
  Sum1/1 -> PI-Control/1(In1)
  Sum/1 -> Sum1/1
  "mQ droop "/1 -> Sum/1
  RMS/1 -> Transfer Fcn2/1
  Demux/2 -> Transfer Fcn/1
  Demux/1 -> Transfer Fcn1/1
  3-phase  Instantaneous  Active & Reactive Power/1 -> Demux/1
  v_meas/1 -> RMS/1, 3-phase  Instantaneous  Active & Reactive Power/1
  PI-Control/1(Out1) -> Vpk/1
  Sum3/1 -> w/1
  E_req/1 -> Sum/2
  " pu convert V"/1 -> Sum1/2
  k/1 -> Pmm/1

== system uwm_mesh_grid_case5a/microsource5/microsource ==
  Vpk : Inport  OutDataType=fixdt(1, 16)  OutScaling=2^0
  w : Inport  Port=2  OutDataType=fixdt(1, 16)  OutScaling=2^0
  Demux : Demux  Outputs=3
  Ground2 : powerlib/Elements/Ground  DialogController=POWERSYS.PowerSysDialog  PhysicalDomain=powersysdomain  SubClassName=unknown  LeftPortType=p1  RightPortType=p1  LConnTagsString=a
  Integrator : Integrator
  Mux : Mux  Inputs=3
  Product : Product  OutDataType=sfix(16)  OutScaling=2^0
  Series RLC Branch : powerlib/Elements/Series RLC Branch  DialogController=POWERSYS.PowerSysDialog  PhysicalDomain=powersysdomain  SubClassName=unknown  LeftPortType=p1  RightPortType=p1  LConnTagsString=__new0  RConnTagsString=__new0  BranchType=C  Resistance=1  Inductance=1e-3  SetiL0=off  InitialCurrent=0  Capacitance=1e-8  Setx0=off  InitialVoltage=0  Measurements=None
  phaseA : powerlib/Electrical Sources/Controlled Voltage Source  DialogController=POWERSYS.PowerSysDialog  SystemSampleTime=-1  Initialize=on  Source_Type=AC  Amplitude=0  Phase=0  Frequency=0  Measurements=None
  phaseB : powerlib/Electrical Sources/Controlled Voltage Source  DialogController=POWERSYS.PowerSysDialog  SystemSampleTime=-1  Initialize=on  Source_Type=AC  Amplitude=0  Phase=0  Frequency=0  Measurements=None
  phaseC : powerlib/Electrical Sources/Controlled Voltage Source  DialogController=POWERSYS.PowerSysDialog  SystemSampleTime=-1  Initialize=on  Source_Type=AC  Amplitude=0  Phase=0  Frequency=0  Measurements=None
  v_A : Fcn  Expr=cos(u)
  v_B : Fcn  Expr=cos(u-2*pi/3)
  v_C : Fcn  Expr=cos(u+2*pi/3)
  Va : PMIOPort  Tag=PMCPort  Port=1  Side=Right
  Vb : PMIOPort  Tag=PMCPort  Port=2  Side=Right
  Vc : PMIOPort  Tag=PMCPort  Port=3  Side=Right
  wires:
  Product/1 -> Demux/1
  Vpk/1 -> Product/1
  Mux/1 -> Product/2
  w/1 -> Integrator/1
  Integrator/1 -> v_A/1, v_B/1, v_C/1
  v_A/1 -> Mux/1
  v_B/1 -> Mux/2
  v_C/1 -> Mux/3
  Demux/1 -> phaseA/1
  Demux/2 -> phaseB/1
  Demux/3 -> phaseC/1
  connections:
  Vb/RConn1 -- phaseB/RConn1 -- phaseA/LConn1
  Va/RConn1 -- phaseC/LConn1 -- phaseA/RConn1
  Vc/RConn1 -- phaseC/RConn1
  Series RLC Branch/RConn1 -- Ground2/LConn1
  Series RLC Branch/LConn1 -- phaseB/LConn1

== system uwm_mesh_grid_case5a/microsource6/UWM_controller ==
  note: P
  note: Q
  v_meas : Inport
  i_meas : Inport  Port=2
  E_req : Inport  Port=3
  P_req : Inport  Port=4
  " pu convert P" : Gain  Gain=1/Sbase  ParameterDataType=sfix(16)  ParameterScaling=2^0  OutDataType=sfix(16)  OutScaling=2^0
  " pu convert S" : Gain  Gain=1/Sbase  ParameterDataType=sfix(16)  ParameterScaling=2^0  OutDataType=sfix(16)  OutScaling=2^0
  " pu convert V" : Gain  Gain=1/(Vbase/sqrt(3))  ParameterDataType=sfix(16)  ParameterScaling=2^0  OutDataType=sfix(16)  OutScaling=2^0
  3-phase  Instantaneous  Active & Reactive Power : powerlib_extras/Measurements/3-phase  Instantaneous  Active & Reactive Power  DialogController=POWERSYS.PowerSysDialog  SystemSampleTime=-1
  Demux : Demux  Outputs=2
  PI-Control : Subsystem
  RMS : Fcn  Expr=sqrt(u(1)*u(1)+u(2)*u(2)+u(3)*u(3))/sqrt(3)
  Sum : Sum  Inputs=|-+  OutDataType=sfix(16)  OutScaling=2^0
  Sum1 : Sum  Inputs=|+-  OutDataType=sfix(16)  OutScaling=2^0
  Sum2 : Sum  Inputs=+-|  OutDataType=sfix(16)  OutScaling=2^0
  Sum3 : Sum  Inputs=+++  OutDataType=sfix(16)  OutScaling=2^0
  Transfer Fcn : TransferFcn  Denominator=[.01 1]
  Transfer Fcn1 : TransferFcn  Denominator=[.01 1]
  Transfer Fcn2 : TransferFcn  Denominator=[.01 1]
  k : Gain  Gain=1/pi  ParameterDataType=sfix(16)  ParameterScaling=2^0  OutDataType=sfix(16)  OutScaling=2^0
  limiter : Subsystem
  mP droop : Gain  Gain=pi  ParameterDataType=sfix(16)  ParameterScaling=2^0  OutDataType=sfix(16)  OutScaling=2^0
  "mQ droop " : Gain  Gain=0.05  ParameterDataType=sfix(16)  ParameterScaling=2^0  OutDataType=sfix(16)  OutScaling=2^0
  w0 : Constant  Value=60*2*pi  OutDataType=fixdt(1, 16)  OutScaling=2^0
  Vpk : Outport
  w : Outport  Port=2
  Pmm : Outport  Port=3
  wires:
  Transfer Fcn2/1 -> " pu convert V"/1
  Transfer Fcn/1 -> " pu convert P"/1
  " pu convert P"/1 -> "mQ droop "/1
  Transfer Fcn1/1 -> " pu convert S"/1
  " pu convert S"/1 -> limiter/1(In1), Sum2/2
  i_meas/1 -> 3-phase  Instantaneous  Active & Reactive Power/2
  P_req/1 -> Sum2/1
  mP droop/1 -> Sum3/2
  limiter/1(Out1) -> Sum3/1, k/1
  w0/1 -> Sum3/3
  Sum2/1 -> mP droop/1
  Sum1/1 -> PI-Control/1(In1)
  Sum/1 -> Sum1/1
  "mQ droop "/1 -> Sum/1
  RMS/1 -> Transfer Fcn2/1
  Demux/2 -> Transfer Fcn/1
  Demux/1 -> Transfer Fcn1/1
  3-phase  Instantaneous  Active & Reactive Power/1 -> Demux/1
  v_meas/1 -> RMS/1, 3-phase  Instantaneous  Active & Reactive Power/1
  PI-Control/1(Out1) -> Vpk/1
  Sum3/1 -> w/1
  E_req/1 -> Sum/2
  " pu convert V"/1 -> Sum1/2
  k/1 -> Pmm/1

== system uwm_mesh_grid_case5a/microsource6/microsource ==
  Vpk : Inport  OutDataType=fixdt(1, 16)  OutScaling=2^0
  w : Inport  Port=2  OutDataType=fixdt(1, 16)  OutScaling=2^0
  Demux : Demux  Outputs=3
  Ground2 : powerlib/Elements/Ground  DialogController=POWERSYS.PowerSysDialog  PhysicalDomain=powersysdomain  SubClassName=unknown  LeftPortType=p1  RightPortType=p1  LConnTagsString=a
  Integrator : Integrator
  Mux : Mux  Inputs=3
  Product : Product  OutDataType=sfix(16)  OutScaling=2^0
  Series RLC Branch : powerlib/Elements/Series RLC Branch  DialogController=POWERSYS.PowerSysDialog  PhysicalDomain=powersysdomain  SubClassName=unknown  LeftPortType=p1  RightPortType=p1  LConnTagsString=__new0  RConnTagsString=__new0  BranchType=C  Resistance=1  Inductance=1e-3  SetiL0=off  InitialCurrent=0  Capacitance=1e-8  Setx0=off  InitialVoltage=0  Measurements=None
  phaseA : powerlib/Electrical Sources/Controlled Voltage Source  DialogController=POWERSYS.PowerSysDialog  SystemSampleTime=-1  Initialize=on  Source_Type=AC  Amplitude=0  Phase=0  Frequency=0  Measurements=None
  phaseB : powerlib/Electrical Sources/Controlled Voltage Source  DialogController=POWERSYS.PowerSysDialog  SystemSampleTime=-1  Initialize=on  Source_Type=AC  Amplitude=0  Phase=0  Frequency=0  Measurements=None
  phaseC : powerlib/Electrical Sources/Controlled Voltage Source  DialogController=POWERSYS.PowerSysDialog  SystemSampleTime=-1  Initialize=on  Source_Type=AC  Amplitude=0  Phase=0  Frequency=0  Measurements=None
  v_A : Fcn  Expr=cos(u)
  v_B : Fcn  Expr=cos(u-2*pi/3)
  v_C : Fcn  Expr=cos(u+2*pi/3)
  Va : PMIOPort  Tag=PMCPort  Port=1  Side=Right
  Vb : PMIOPort  Tag=PMCPort  Port=2  Side=Right
  Vc : PMIOPort  Tag=PMCPort  Port=3  Side=Right
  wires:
  Product/1 -> Demux/1
  Vpk/1 -> Product/1
  Mux/1 -> Product/2
  w/1 -> Integrator/1
  Integrator/1 -> v_A/1, v_B/1, v_C/1
  v_A/1 -> Mux/1
  v_B/1 -> Mux/2
  v_C/1 -> Mux/3
  Demux/1 -> phaseA/1
  Demux/2 -> phaseB/1
  Demux/3 -> phaseC/1
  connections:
  Vb/RConn1 -- phaseB/RConn1 -- phaseA/LConn1
  Va/RConn1 -- phaseC/LConn1 -- phaseA/RConn1
  Vc/RConn1 -- phaseC/RConn1
  Series RLC Branch/RConn1 -- Ground2/LConn1
  Series RLC Branch/LConn1 -- phaseB/LConn1

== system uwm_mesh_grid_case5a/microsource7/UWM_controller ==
  note: P
  note: Q
  v_meas : Inport
  i_meas : Inport  Port=2
  E_req : Inport  Port=3
  P_req : Inport  Port=4
  " pu convert P" : Gain  Gain=1/Sbase  ParameterDataType=sfix(16)  ParameterScaling=2^0  OutDataType=sfix(16)  OutScaling=2^0
  " pu convert S" : Gain  Gain=1/Sbase  ParameterDataType=sfix(16)  ParameterScaling=2^0  OutDataType=sfix(16)  OutScaling=2^0
  " pu convert V" : Gain  Gain=1/(Vbase/sqrt(3))  ParameterDataType=sfix(16)  ParameterScaling=2^0  OutDataType=sfix(16)  OutScaling=2^0
  3-phase  Instantaneous  Active & Reactive Power : powerlib_extras/Measurements/3-phase  Instantaneous  Active & Reactive Power  DialogController=POWERSYS.PowerSysDialog  SystemSampleTime=-1
  Demux : Demux  Outputs=2
  PI-Control : Subsystem
  RMS : Fcn  Expr=sqrt(u(1)*u(1)+u(2)*u(2)+u(3)*u(3))/sqrt(3)
  Sum : Sum  Inputs=|-+  OutDataType=sfix(16)  OutScaling=2^0
  Sum1 : Sum  Inputs=|+-  OutDataType=sfix(16)  OutScaling=2^0
  Sum2 : Sum  Inputs=+-|  OutDataType=sfix(16)  OutScaling=2^0
  Sum3 : Sum  Inputs=+++  OutDataType=sfix(16)  OutScaling=2^0
  Transfer Fcn : TransferFcn  Denominator=[.01 1]
  Transfer Fcn1 : TransferFcn  Denominator=[.01 1]
  Transfer Fcn2 : TransferFcn  Denominator=[.01 1]
  k : Gain  Gain=1/pi  ParameterDataType=sfix(16)  ParameterScaling=2^0  OutDataType=sfix(16)  OutScaling=2^0
  limiter : Subsystem
  mP droop : Gain  Gain=pi  ParameterDataType=sfix(16)  ParameterScaling=2^0  OutDataType=sfix(16)  OutScaling=2^0
  "mQ droop " : Gain  Gain=0.05  ParameterDataType=sfix(16)  ParameterScaling=2^0  OutDataType=sfix(16)  OutScaling=2^0
  w0 : Constant  Value=60*2*pi  OutDataType=fixdt(1, 16)  OutScaling=2^0
  Vpk : Outport
  w : Outport  Port=2
  Pmm : Outport  Port=3
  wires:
  Transfer Fcn2/1 -> " pu convert V"/1
  Transfer Fcn/1 -> " pu convert P"/1
  " pu convert P"/1 -> "mQ droop "/1
  Transfer Fcn1/1 -> " pu convert S"/1
  " pu convert S"/1 -> limiter/1(In1), Sum2/2
  i_meas/1 -> 3-phase  Instantaneous  Active & Reactive Power/2
  P_req/1 -> Sum2/1
  mP droop/1 -> Sum3/2
  limiter/1(Out1) -> Sum3/1, k/1
  w0/1 -> Sum3/3
  Sum2/1 -> mP droop/1
  Sum1/1 -> PI-Control/1(In1)
  Sum/1 -> Sum1/1
  "mQ droop "/1 -> Sum/1
  RMS/1 -> Transfer Fcn2/1
  Demux/2 -> Transfer Fcn/1
  Demux/1 -> Transfer Fcn1/1
  3-phase  Instantaneous  Active & Reactive Power/1 -> Demux/1
  v_meas/1 -> RMS/1, 3-phase  Instantaneous  Active & Reactive Power/1
  PI-Control/1(Out1) -> Vpk/1
  Sum3/1 -> w/1
  E_req/1 -> Sum/2
  " pu convert V"/1 -> Sum1/2
  k/1 -> Pmm/1

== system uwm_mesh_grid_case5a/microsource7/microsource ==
  Vpk : Inport  OutDataType=fixdt(1, 16)  OutScaling=2^0
  w : Inport  Port=2  OutDataType=fixdt(1, 16)  OutScaling=2^0
  Demux : Demux  Outputs=3
  Ground2 : powerlib/Elements/Ground  DialogController=POWERSYS.PowerSysDialog  PhysicalDomain=powersysdomain  SubClassName=unknown  LeftPortType=p1  RightPortType=p1  LConnTagsString=a
  Integrator : Integrator
  Mux : Mux  Inputs=3
  Product : Product  OutDataType=sfix(16)  OutScaling=2^0
  Series RLC Branch : powerlib/Elements/Series RLC Branch  DialogController=POWERSYS.PowerSysDialog  PhysicalDomain=powersysdomain  SubClassName=unknown  LeftPortType=p1  RightPortType=p1  LConnTagsString=__new0  RConnTagsString=__new0  BranchType=C  Resistance=1  Inductance=1e-3  SetiL0=off  InitialCurrent=0  Capacitance=1e-8  Setx0=off  InitialVoltage=0  Measurements=None
  phaseA : powerlib/Electrical Sources/Controlled Voltage Source  DialogController=POWERSYS.PowerSysDialog  SystemSampleTime=-1  Initialize=on  Source_Type=AC  Amplitude=0  Phase=0  Frequency=0  Measurements=None
  phaseB : powerlib/Electrical Sources/Controlled Voltage Source  DialogController=POWERSYS.PowerSysDialog  SystemSampleTime=-1  Initialize=on  Source_Type=AC  Amplitude=0  Phase=0  Frequency=0  Measurements=None
  phaseC : powerlib/Electrical Sources/Controlled Voltage Source  DialogController=POWERSYS.PowerSysDialog  SystemSampleTime=-1  Initialize=on  Source_Type=AC  Amplitude=0  Phase=0  Frequency=0  Measurements=None
  v_A : Fcn  Expr=cos(u)
  v_B : Fcn  Expr=cos(u-2*pi/3)
  v_C : Fcn  Expr=cos(u+2*pi/3)
  Va : PMIOPort  Tag=PMCPort  Port=1  Side=Right
  Vb : PMIOPort  Tag=PMCPort  Port=2  Side=Right
  Vc : PMIOPort  Tag=PMCPort  Port=3  Side=Right
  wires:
  Product/1 -> Demux/1
  Vpk/1 -> Product/1
  Mux/1 -> Product/2
  w/1 -> Integrator/1
  Integrator/1 -> v_A/1, v_B/1, v_C/1
  v_A/1 -> Mux/1
  v_B/1 -> Mux/2
  v_C/1 -> Mux/3
  Demux/1 -> phaseA/1
  Demux/2 -> phaseB/1
  Demux/3 -> phaseC/1
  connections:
  Vb/RConn1 -- phaseB/RConn1 -- phaseA/LConn1
  Va/RConn1 -- phaseC/LConn1 -- phaseA/RConn1
  Vc/RConn1 -- phaseC/RConn1
  Series RLC Branch/RConn1 -- Ground2/LConn1
  Series RLC Branch/LConn1 -- phaseB/LConn1

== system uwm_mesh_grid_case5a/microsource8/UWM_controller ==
  note: P
  note: Q
  v_meas : Inport
  i_meas : Inport  Port=2
  E_req : Inport  Port=3
  P_req : Inport  Port=4
  " pu convert P" : Gain  Gain=1/Sbase  ParameterDataType=sfix(16)  ParameterScaling=2^0  OutDataType=sfix(16)  OutScaling=2^0
  " pu convert S" : Gain  Gain=1/Sbase  ParameterDataType=sfix(16)  ParameterScaling=2^0  OutDataType=sfix(16)  OutScaling=2^0
  " pu convert V" : Gain  Gain=1/(Vbase/sqrt(3))  ParameterDataType=sfix(16)  ParameterScaling=2^0  OutDataType=sfix(16)  OutScaling=2^0
  3-phase  Instantaneous  Active & Reactive Power : powerlib_extras/Measurements/3-phase  Instantaneous  Active & Reactive Power  DialogController=POWERSYS.PowerSysDialog  SystemSampleTime=-1
  Demux : Demux  Outputs=2
  PI-Control : Subsystem
  RMS : Fcn  Expr=sqrt(u(1)*u(1)+u(2)*u(2)+u(3)*u(3))/sqrt(3)
  Sum : Sum  Inputs=|-+  OutDataType=sfix(16)  OutScaling=2^0
  Sum1 : Sum  Inputs=|+-  OutDataType=sfix(16)  OutScaling=2^0
  Sum2 : Sum  Inputs=+-|  OutDataType=sfix(16)  OutScaling=2^0
  Sum3 : Sum  Inputs=+++  OutDataType=sfix(16)  OutScaling=2^0
  Transfer Fcn : TransferFcn  Denominator=[.01 1]
  Transfer Fcn1 : TransferFcn  Denominator=[.01 1]
  Transfer Fcn2 : TransferFcn  Denominator=[.01 1]
  k : Gain  Gain=1/pi  ParameterDataType=sfix(16)  ParameterScaling=2^0  OutDataType=sfix(16)  OutScaling=2^0
  limiter : Subsystem
  mP droop : Gain  Gain=pi  ParameterDataType=sfix(16)  ParameterScaling=2^0  OutDataType=sfix(16)  OutScaling=2^0
  "mQ droop " : Gain  Gain=0.05  ParameterDataType=sfix(16)  ParameterScaling=2^0  OutDataType=sfix(16)  OutScaling=2^0
  w0 : Constant  Value=60*2*pi  OutDataType=fixdt(1, 16)  OutScaling=2^0
  Vpk : Outport
  w : Outport  Port=2
  Pmm : Outport  Port=3
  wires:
  Transfer Fcn2/1 -> " pu convert V"/1
  Transfer Fcn/1 -> " pu convert P"/1
  " pu convert P"/1 -> "mQ droop "/1
  Transfer Fcn1/1 -> " pu convert S"/1
  " pu convert S"/1 -> limiter/1(In1), Sum2/2
  i_meas/1 -> 3-phase  Instantaneous  Active & Reactive Power/2
  P_req/1 -> Sum2/1
  mP droop/1 -> Sum3/2
  limiter/1(Out1) -> Sum3/1, k/1
  w0/1 -> Sum3/3
  Sum2/1 -> mP droop/1
  Sum1/1 -> PI-Control/1(In1)
  Sum/1 -> Sum1/1
  "mQ droop "/1 -> Sum/1
  RMS/1 -> Transfer Fcn2/1
  Demux/2 -> Transfer Fcn/1
  Demux/1 -> Transfer Fcn1/1
  3-phase  Instantaneous  Active & Reactive Power/1 -> Demux/1
  v_meas/1 -> RMS/1, 3-phase  Instantaneous  Active & Reactive Power/1
  PI-Control/1(Out1) -> Vpk/1
  Sum3/1 -> w/1
  E_req/1 -> Sum/2
  " pu convert V"/1 -> Sum1/2
  k/1 -> Pmm/1
